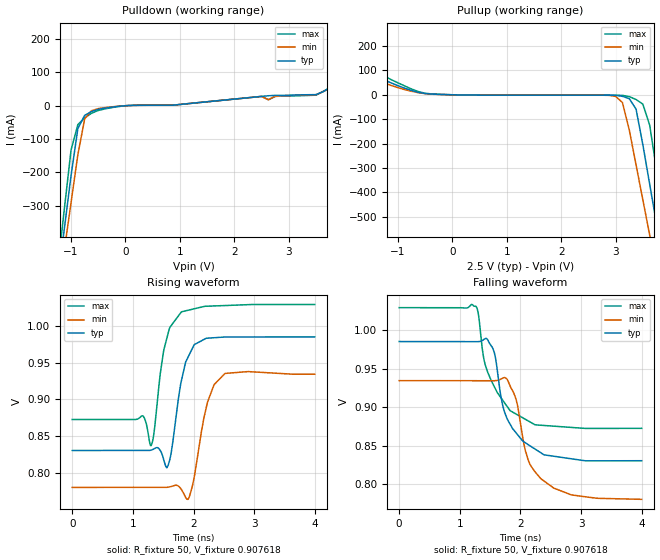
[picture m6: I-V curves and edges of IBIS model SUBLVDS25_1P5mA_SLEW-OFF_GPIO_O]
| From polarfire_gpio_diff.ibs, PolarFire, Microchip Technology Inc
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|   Model SUBLVDS25_1P5mA_SLEW-OFF_GPIO_O
[Model]   SUBLVDS25_1P5mA_SLEW-OFF_GPIO_O
Model_type   Output
Polarity   Non-Inverting
Enable   Active-High
Vmeas =   0.9
Cref =   5p
Rref =   100
|   typ   min   max
C_comp_pullup   2.605e-12   2.605e-12   2.76e-12
C_comp_pulldown  2.605e-12   2.605e-12   2.76e-12
[Temperature Range]  25C   100C   -40C
[Voltage Range]  2.5   2.375   2.625
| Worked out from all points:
|   slope of the pulldown table from 0 to 0.375 V, typ, clamps not added: 270 ohm
|   slope of the pullup table from 0 to 0.375 V, typ, clamps not added: 279 ohm
|   rising waveform, R_fixture 50, V_fixture 0.907618: 20-80 % time 202ps typ, 218ps min, 198ps max; typ from 0.831 V to 0.985 V
|   falling waveform, R_fixture 50, V_fixture 0.907618: 20-80 % time 375ps typ, 344ps min, 413ps max; typ from 0.985 V to 0.831 V
[Pulldown]
|Voltage   I(typ)   I(min)   I(max)
-2.5V     -2.163A    -2.026A    -2.344A
-1.25V    -533mA     -578.6mA   -495.5mA
-1.125V   -371.3mA   -434.8mA   -312.4mA
-1V       -209.8mA   -290.9mA   -133.1mA
-875mV    -68.69mA   -147.3mA   -56.88mA
-750mV    -29.01mA   -39.74mA   -36.89mA
-625mV    -17.57mA   -14.99mA   -22.64mA
0V        -44.43uA   -37.95uA   -54.54uA
875mV     1.558mA    1.575mA    1.55mA
3.5V      33.19mA    32.64mA    31.52mA
4.125V    92.46mA    86.19mA    98.29mA
5V        211.3mA    189.5mA    234mA
[Pullup]
|Voltage   I(typ)   I(min)   I(max)
-2.5V     228.6mA    189mA      273.5mA
-500mV    5.241mA    4.698mA    6.228mA
3V        -2.282mA   -6.556mA   -1.662mA
3.125V    -6.22mA    -31.76mA   -2.46mA
3.25V     -15.87mA   -143.6mA   -7.341mA
3.375V    -58.6mA    -287.1mA   -19.32mA
3.5V      -204.7mA   -430.7mA   -38.23mA
3.625V    -366mA     -574.3mA   -124.2mA
3.75V     -527.5mA   -717.9mA   -305.7mA
3.875V    -689.2mA   -861.6mA   -488.5mA
4V        -851mA     -1.005A    -671.4mA
5V        -2.155A    -2.167A    -2.147A
[Ramp]
| variable   typ   min   max
dV/dt_r 0.1068/0.2069e-9   0.1043/0.2406e-9   0.1152/0.4675e-9
dV/dt_f 95.3703e-3/0.3728e-9   94.8718e-3/0.3458e-9   96.5446e-3/0.4109e-9
R_load = 50
[Rising waveform]
R_fixture= 50
V_fixture= 0.907618
V_fixture_min= 0.856988
V_fixture_max= 0.950984
|Time   V(typ)   V(min)   V(max)
0s        830.6mV    780.4mV    872.7mV
1.16ns    830.6mV    780.4mV    877.8mV
1.3ns     831.1mV    780.4mV    837.2mV
1.5ns     820.7mV    780.3mV    962.3mV
1.58ns    810.1mV    780.7mV    989.5mV
1.79ns    921.8mV    778.9mV    1.018V
1.91ns    957.6mV    764.2mV    1.021V
2.23ns    983.3mV    896mV      1.027V
2.52ns    984.9mV    935.4mV    1.028V
4ns       985.1mV    934.4mV    1.029V
[Falling waveform]
R_fixture= 50
V_fixture= 0.907618
V_fixture_min= 0.856988
V_fixture_max= 0.950984
|Time   V(typ)   V(min)   V(max)
0s        985.1mV    934.4mV    1.029V
1.27ns    984.9mV    934.4mV    1.031V
1.4ns     988mV      934.4mV    961.5mV
1.55ns    975.3mV    934.2mV    929.7mV
1.75ns    891.3mV    938.2mV    904.2mV
1.93ns    866.6mV    909.8mV    891.1mV
2.13ns    851.3mV    831.2mV    882.1mV
2.33ns    841mV      807.8mV    876.6mV
2.84ns    833mV      786.2mV    873.7mV
4ns       830.5mV    780.4mV    872.6mV
